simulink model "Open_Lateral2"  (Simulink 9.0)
settings: Solver=ode45  StartTime=0.0  StopTime=100  RelTol=1e-3  EnableMultiTasking=on
InitFcn:
  | init_lat;
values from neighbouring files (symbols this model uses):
  Cyb = -0.023    [init_lat.m]    (also in init.m; init_pitch.m)
  Cyda = 0.0011    [init_lat.m]    (also in init.m; init_pitch.m)
  Cydr = 0.0034    [init_lat.m]    (also in init.m; init_pitch.m)
  d2r = pi/180    (= 0.0174532925199)    [frequ.m]    (also in init_lat.m; pl.m; init.m; freq.m)
  Mv = 1219.1    [init_lat.m]    (also in init.m; init_pitch.m)
  Qbar = 1220.6    [init_lat.m]    (also in init.m; init_pitch.m)
  Sref = 145.4    [init_lat.m]    (also in init.m; init_pitch.m)
undefined symbols (not defined in the file or in its folder): Al, Bl, Cl, Dl, Kpr

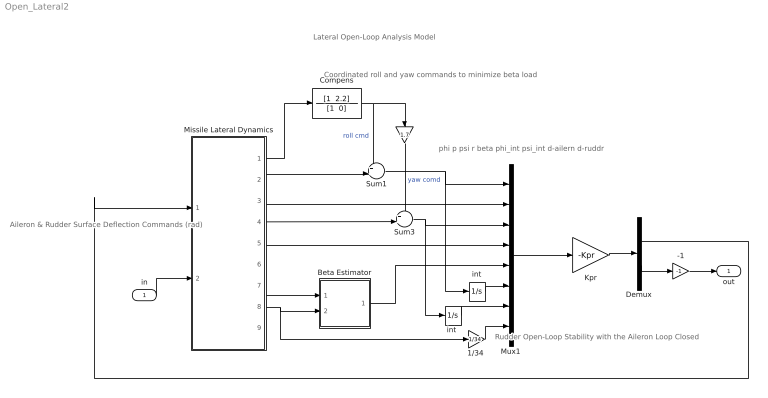
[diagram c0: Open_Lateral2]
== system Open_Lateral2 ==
  note: phi p psi r beta phi_int psi_int d-ailern d-ruddr
  note: Aileron & Rudder Surface Deflection Commands (rad)
  note: Coordinated roll and yaw commands to minimize beta load
  note: Lateral Open-Loop Analysis Model
  note: Rudder Open-Loop Stability with the Aileron Loop Closed
  in : Inport
  " " : Gain  Gain=1.7
  -1 : Gain  Gain=-1
  "1/34 " : Gain  Gain=1/34
  Beta Estimator : Subsystem
  Compens : TransferFcn  Numerator="[1  2.2]"  Denominator="[1  0]"
  Demux : Demux  Outputs=2
  Kpr : Gain  Gain=-Kpr  Multiplication=Matrix(K*u)
  Missile Lateral Dynamics : Subsystem
  Mux1 : Mux  Inputs=[1, 1, 1, 1, 1, 1, 1, 2]
  Sum1 : Sum  Inputs=++|
  Sum3 : Sum  Inputs=++|
  int : Integrator
  "int " : Integrator
  out : Outport
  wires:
  Missile Lateral Dynamics/3(p) -> Mux1/2
  Missile Lateral Dynamics/5(r) -> Mux1/4
  Sum1/1 -> Mux1/1, int/1
  Missile Lateral Dynamics/2(phi) -> Sum1/2
  Missile Lateral Dynamics/1(" Head") -> Compens/1
  int/1 -> Mux1/6
  Compens/1 -> " "/1, Sum1/1  "roll cmd"
  Missile Lateral Dynamics/4(psi) -> Sum3/2
  Sum3/1 -> Mux1/3, "int "/1
  "int "/1 -> Mux1/7
  " "/1 -> Sum3/1  "yaw comd"
  Missile Lateral Dynamics/8(aeros) -> Beta Estimator/2(delta), "1/34 "/1
  Mux1/1 -> Kpr/1
  Kpr/1 -> Demux/1
  -1/1 -> out/1
  "1/34 "/1 -> Mux1/8
  Missile Lateral Dynamics/7(Ny) -> Beta Estimator/1(Ny)
  Beta Estimator/1(beta) -> Mux1/5
  Demux/2 -> -1/1
  in/1 -> Missile Lateral Dynamics/2(ruddr)
  Demux/1 -> Missile Lateral Dynamics/1(ailer)

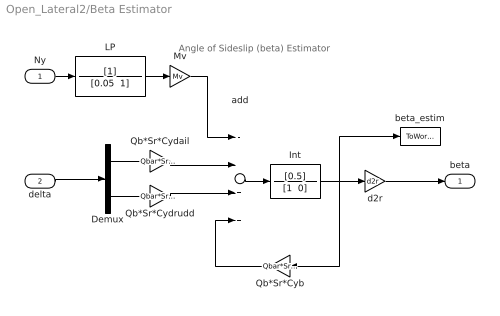
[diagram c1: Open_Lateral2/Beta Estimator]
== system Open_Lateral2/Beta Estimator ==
  note: Angle of Sideslip (beta) Estimator
  Ny : Inport
  delta : Inport  Port=2
  Demux : Demux  Outputs=2
  Int : TransferFcn  Numerator=[0.5]  Denominator="[1  0]"
  LP : TransferFcn  Denominator="[0.05  1]"
  Mv : Gain  Gain=Mv
  Qb*Sr*Cyb : Gain  Gain=Qbar*Sref*Cyb*1.2
  Qb*Sr*Cydail : Gain  Gain=Qbar*Sref*Cyda
  Qb*Sr*Cydrudd : Gain  Gain=Qbar*Sref*Cydr
  add : Sum  Inputs=-+++
  beta_estim : ToWorkspace  VariableName=beta_vn  SampleTime=-1
  d2r : Gain  Gain=d2r
  beta : Outport
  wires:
  LP/1 -> Mv/1
  Qb*Sr*Cydail/1 -> add/2
  Qb*Sr*Cydrudd/1 -> add/3
  Qb*Sr*Cyb/1 -> add/4
  Ny/1 -> LP/1
  Int/1 -> beta_estim/1, d2r/1, Qb*Sr*Cyb/1
  d2r/1 -> beta/1
  Mv/1 -> add/1
  add/1 -> Int/1
  Demux/1 -> Qb*Sr*Cydail/1
  Demux/2 -> Qb*Sr*Cydrudd/1
  delta/1 -> Demux/1

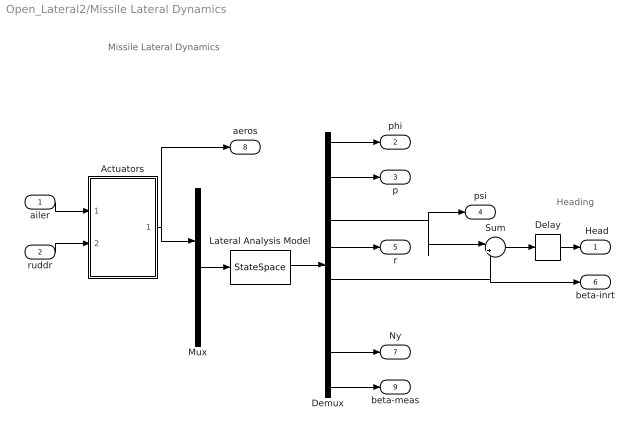
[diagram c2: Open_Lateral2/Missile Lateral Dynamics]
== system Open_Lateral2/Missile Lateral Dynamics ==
  note: Heading
  note: Missile Lateral Dynamics
  ailer : Inport
  ruddr : Inport  Port=2
  Actuators : Subsystem
  Delay : TransportDelay  DelayTime=0.5  PadeOrder=2
  Demux : Demux  Outputs=8
  Lateral Analysis Model : StateSpace  A=Al  B=Bl  C=Cl  D=Dl  InitialCondition=0
  Mux : Mux  Inputs=[2, 1]
  Sum : Sum  Inputs=|++
  " Head" : Outport
  phi : Outport  Port=2
  p : Outport  Port=3
  psi : Outport  Port=4
  r : Outport  Port=5
  beta-inrt : Outport  Port=6
  Ny : Outport  Port=7
  aeros : Outport  Port=8
  beta-meas : Outport  Port=9
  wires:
  Mux/1 -> Lateral Analysis Model/1
  Demux/1 -> phi/1
  Demux/2 -> p/1
  Demux/4 -> r/1
  Demux/3 -> psi/1, Sum/1
  Demux/5 -> beta-inrt/1, Sum/2
  Actuators/1("delo ") -> aeros/1, Mux/1
  Sum/1 -> Delay/1
  ailer/1 -> Actuators/1(dailer)
  ruddr/1 -> Actuators/2(drudr)
  Demux/7 -> Ny/1
  Demux/8 -> beta-meas/1
  Lateral Analysis Model/1 -> Demux/1
  Delay/1 -> " Head"/1

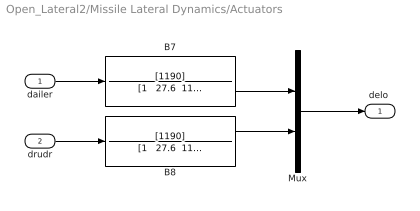
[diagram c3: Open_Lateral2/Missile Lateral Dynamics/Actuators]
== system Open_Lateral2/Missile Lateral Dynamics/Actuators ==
  dailer : Inport
  drudr : Inport  Port=2
  B7 : TransferFcn  Numerator=[1190]  Denominator="[1   27.6  1190]"
  B8 : TransferFcn  Numerator=[1190]  Denominator="[1   27.6  1190]"
  Mux : Mux  Inputs=2
  "delo " : Outport
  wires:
  Mux/1 -> "delo "/1
  B7/1 -> Mux/1
  B8/1 -> Mux/2
  drudr/1 -> B8/1
  dailer/1 -> B7/1
